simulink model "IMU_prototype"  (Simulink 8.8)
settings: Solver=ode45  StartTime=0.0  StopTime=1  RelTol=1e-3  EnableMultiTasking=on

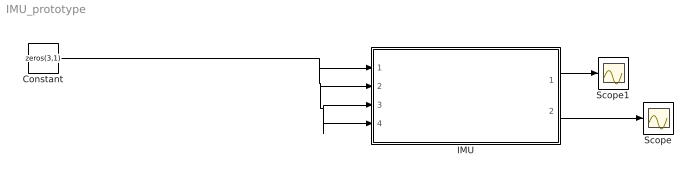
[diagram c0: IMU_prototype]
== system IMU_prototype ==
  Constant : Constant  Value=zeros(3,1)  SampleTime=0
  IMU : Subsystem
  Scope : Scope
  Scope1 : Scope
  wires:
  IMU/1(accelerometer) -> Scope1/1
  Constant/1 -> IMU/4(B_Fg), IMU/3(B_Omega), IMU/2(B_vo), IMU/1(B_vo_dot)
  IMU/2(gyroscope) -> Scope/1

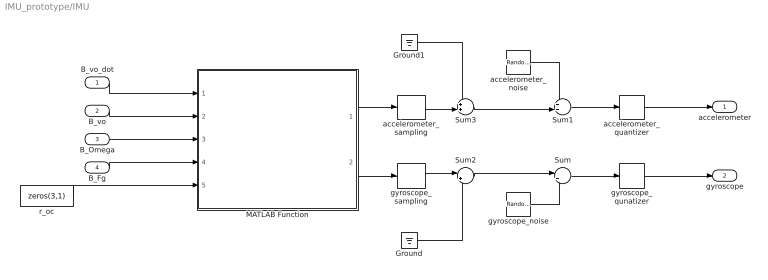
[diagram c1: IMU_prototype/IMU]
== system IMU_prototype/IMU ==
  B_vo_dot : Inport
  B_vo : Inport  Port=2
  B_Omega : Inport  Port=3
  B_Fg : Inport  Port=4
  Ground : Ground
  Ground1 : Ground
  MATLAB Function : MATLAB Function  TreatAsAtomicUnit=on
  Sum : Sum  Inputs=|++
  Sum1 : Sum  Inputs=++|
  Sum2 : Sum  Inputs=|++
  Sum3 : Sum  Inputs=++|
  accelerometer_noise : RandomNumber  Mean=zeros(3,1)  Variance=[ 3e-7 ; 3.3e-7 ; 7.2e-7 ]  Seed=[0,1,2]  SampleTime=6.1e-3
  accelerometer_quantizer : Quantizer  QuantizationInterval=2.4400e-04
  accelerometer_sampling : ZeroOrderHold  SampleTime=6.1e-3
  gyroscope_noise : RandomNumber  Mean=zeros(3,1)  Variance=[ 2.2e-8 ; 1.1e-7 ; 2.4e-8 ]  Seed=[0,1,2]  SampleTime=6.1e-3
  gyroscope_qunatizer : Quantizer  QuantizationInterval=1.1e-3
  gyroscope_sampling : ZeroOrderHold  SampleTime=6.1e-3
  r_oc : Constant  Value=zeros(3,1)
  accelerometer : Outport
  gyroscope : Outport  Port=2
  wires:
  gyroscope_qunatizer/1 -> gyroscope/1
  accelerometer_quantizer/1 -> accelerometer/1
  accelerometer_noise/1 -> Sum1/1
  Sum/1 -> gyroscope_qunatizer/1
  Sum2/1 -> Sum/1
  Sum3/1 -> Sum1/2
  MATLAB Function/2(gyro_reading) -> gyroscope_sampling/1
  gyroscope_noise/1 -> Sum/2
  MATLAB Function/1(accel_reading) -> accelerometer_sampling/1
  Sum1/1 -> accelerometer_quantizer/1
  gyroscope_sampling/1 -> Sum2/1
  accelerometer_sampling/1 -> Sum3/2
  Ground/1 -> Sum2/2
  Ground1/1 -> Sum3/1
  B_vo_dot/1 -> MATLAB Function/1(B_vo_dot)
  B_vo/1 -> MATLAB Function/2(B_vo)
  B_Omega/1 -> MATLAB Function/3(B_Omega)
  B_Fg/1 -> MATLAB Function/4(B_Fg)
  r_oc/1 -> MATLAB Function/5(r_oc)

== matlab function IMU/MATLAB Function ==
function [accel_reading,gyro_reading] = fcn(B_vo_dot, B_vo, B_Omega, B_Fg, r_oc)
%#codegen

a = B_vo_dot + cross(B_Omega,B_vo) ; % body frame acceleration 

accel_reading = a - B_Fg ; % accelerometer reading (ideal)

gyro_reading = B_Omega ; % gyroscope reading (ideal) 

end
